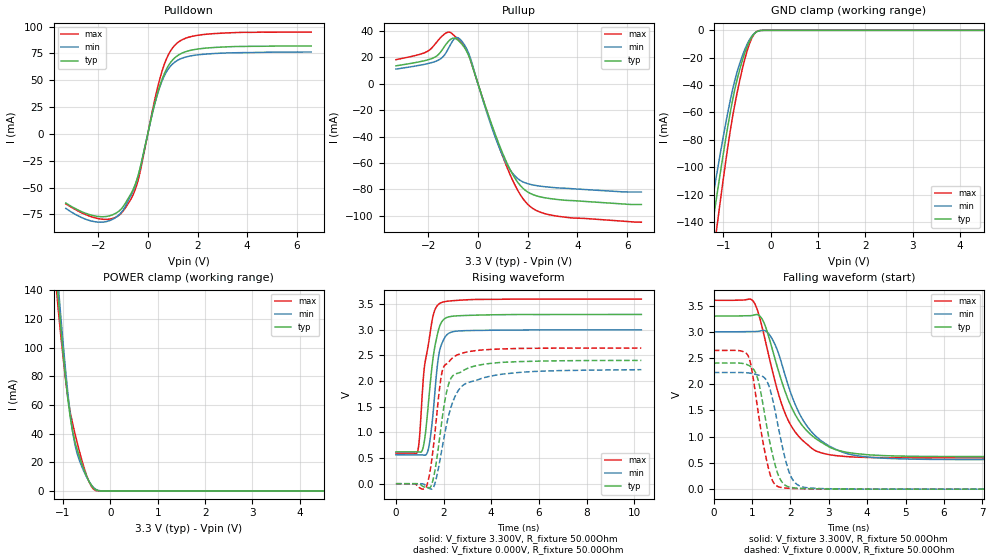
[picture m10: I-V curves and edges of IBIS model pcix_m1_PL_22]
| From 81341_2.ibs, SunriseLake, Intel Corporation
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[Model]   pcix_m1_PL_22
Model_type   I/O
Vinl = 1.155V
Vinh = 1.650V
Vmeas = 1.320V
Vref = 0.000V
Cref = 10.000pF
Rref = 25.000Ohm
|   typ   min   max
C_comp   7.500pF   6.000pF   9.000pF
[Voltage Range]   3.300V   3.000V   3.600V
[Temperature Range]   60.0   110.0   -5.0
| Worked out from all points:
|   slope of the pulldown table from 0 to 0.495 V, typ, clamps not added: 10.9 ohm
|   slope of the pullup table from 0 to 0.495 V, typ, clamps not added: 17.8 ohm
|   GND clamp passes 1 mA (typ) near -0.30 V on its own axis
|   POWER clamp passes 1 mA (typ) near -0.32 V on its own axis
|   falling waveform, V_fixture 3.300V, R_fixture 50.00Ohm: 20-80 % time 884ps typ, 883ps min, 737ps max; typ from 3.3 V to 0.62 V
|   rising waveform, V_fixture 3.300V, R_fixture 50.00Ohm: 20-80 % time 393ps typ, 315ps min, 421ps max; typ from 0.62 V to 3.3 V
|   rising waveform, V_fixture 0.000V, R_fixture 50.00Ohm: 20-80 % time 485ps typ, 727ps min, 388ps max; typ from 0 V to 2.4 V
|   falling waveform, V_fixture 0.000V, R_fixture 50.00Ohm: 20-80 % time 388ps typ, 399ps min, 356ps max; typ from 2.4 V to 0 V
[Pulldown]
|   Voltage   I(typ)   I(min)   I(max)
-3.3V     -64.47mA   -69.44mA   -65.21mA
-1.9V     -77.17mA   -82.31mA   -79.35mA
-1.35V    -74.74mA   -78.78mA   -78.28mA
-950mV    -66.39mA   -69.46mA   -70.57mA
-600mV    -52.29mA   -53.64mA   -57.12mA
-400mV    -39.68mA   -40.38mA   -43.96mA
200mV     20.68mA    20.76mA    23.27mA
500mV     45.92mA    44.9mA     52.67mA
850mV     64.34mA    61.31mA    74.75mA
1.25V     73.73mA    69.22mA    85.88mA
2.65V     80.49mA    74.87mA    93.43mA
6.575V    81.96mA    76.32mA    94.87mA
[GND Clamp]
|   Voltage   I(typ)   I(min)   I(max)
-3.3V     -632.5mA   -564.4mA   -725.5mA
-1.325V   -165.6mA   -144.4mA   -196mA
-1.3V     -159.5mA   -139mA     -189mA
-1.25V    -147.6mA   -128.4mA   -175.3mA
-1.2V     -135.8mA   -118mA     -161.6mA
-1.125V   -118.5mA   -102.6mA   -141.4mA
-850mV    -59.64mA   -50.8mA    -72.97mA
-650mV    -28.41mA   -23.93mA   -36.31mA
-450mV    -8.219mA   -7.112mA   -10.14mA
-350mV    -2.584mA   -2.413mA   -2.802mA
-250mV    -331.3uA   -398.2uA   -220.5uA
6.575V    0A         0A         0A
[Pullup]
|   Voltage   I(typ)   I(min)   I(max)
-3.3V     13.5mA     11.03mA    18.15mA
-2.15V    17.38mA    14.64mA    23.38mA
-1.65V    21.08mA    17.31mA    31.67mA
-1.1V     33.54mA    29.73mA    38.7mA
-850mV    33.56mA    34.9mA     34.67mA
-500mV    26.01mA    27.99mA    26.71mA
500mV     -28.04mA   -29.95mA   -28.73mA
1V        -52.86mA   -54.63mA   -55.12mA
1.5V      -71.83mA   -70.04mA   -77.08mA
2V        -81.86mA   -75.62mA   -91.14mA
3.2V      -87.59mA   -78.79mA   -100.2mA
6.575V    -91.38mA   -81.92mA   -104.7mA
[POWER Clamp]
|   Voltage   I(typ)   I(min)   I(max)
-3.3V     1.109A     1.089A     1.13A
-1.125V   144.6mA    153.4mA    135.7mA
-1.1V     134.6mA    143.1mA    126.5mA
-1.075V   125mA      133.1mA    118mA
-900mV    64.86mA    68.99mA    65.55mA
-800mV    41.99mA    41.86mA    47.4mA
-750mV    34.63mA    32.54mA    40.32mA
-650mV    23.51mA    20.95mA    27.23mA
-500mV    10.16mA    9.585mA    10.63mA
-400mV    3.792mA    4.116mA    3.102mA
-300mV    590.1uA    959uA      205.5uA
6.575V    0A         0A         0A
[Ramp]
R_load = 50.00Ohm
|   typ   min   max
dV/dt_r   1.442V/484.758ps   1.334V/725.060ps   1.587V/387.232ps
dV/dt_f   1.608V/883.635ps   1.462V/882.649ps   1.803V/736.686ps
[Falling Waveform]
V_fixture = 3.300V
V_fixture_min = 3.000V
V_fixture_max = 3.600V
R_fixture = 50.00Ohm
|   Time   V(typ)   V(min)   V(max)
0s        3.3V       3V         3.6V
1.04ns    3.317V     3.004V     3.572V
1.25ns    3.254V     3.023V     3.119V
1.45ns    2.863V     2.947V     2.495V
1.88ns    1.822V     2.122V     1.41V
2.26ns    1.261V     1.403V     970.4mV
2.7ns     943mV      983mV      717.7mV
3.4ns     712.6mV    692.8mV    624.5mV
4.14ns    649.9mV    603.9mV    602.4mV
10.3ns    620.3mV    563mV      595.4mV
[Rising Waveform]
V_fixture = 3.300V
V_fixture_min = 3.000V
V_fixture_max = 3.600V
R_fixture = 50.00Ohm
|   Time   V(typ)   V(min)   V(max)
0s        620.3mV    563mV      595.4mV
900ps     620.3mV    562.4mV    612.8mV
990ps     617.2mV    562.7mV    905.6mV
1.12ns    667mV      561.2mV    1.855V
1.21ns    881.7mV    555.4mV    2.327V
1.41ns    1.804V     792.2mV    2.859V
1.6ns     2.58V      1.585V     3.342V
1.84ns    3.077V     2.606V     3.516V
2.57ns    3.273V     2.976V     3.575V
10.3ns    3.3V       3V         3.6V
[Rising Waveform]
V_fixture = 0.000V
V_fixture_min = 0.000V
V_fixture_max = 0.000V
R_fixture = 50.00Ohm
|   Time   V(typ)   V(min)   V(max)
0s        601.5nV    3.438uV    42.63nV
1.27ns    -72.21mV   -43.87mV   -65.04mV
1.56ns    80.99mV    -85.65mV   671mV
1.82ns    841.2mV    390.1mV    1.814V
1.94ns    1.267V     698.5mV    2.187V
2.2ns     1.924V     1.304V     2.361V
2.5ns     2.139V     1.72V      2.494V
2.95ns    2.238V     1.957V     2.565V
4.35ns    2.362V     2.128V     2.626V
10.3ns    2.404V     2.223V     2.645V
[Falling Waveform]
V_fixture = 0.000V
V_fixture_min = 0.000V
V_fixture_max = 0.000V
R_fixture = 50.00Ohm
|   Time   V(typ)   V(min)   V(max)
0s        2.404V     2.223V     2.645V
900ps     2.363V     2.215V     2.535V
990ps     2.318V     2.206V     2.286V
1.14ns    2.12V      2.178V     1.555V
1.38ns    1.205V     2.064V     544.4mV
1.52ns    697.4mV    1.758V     179.3mV
1.7ns     237.5mV    1.119V     42.69mV
2ns       35.15mV    260.3mV    14.72mV
2.37ns    12.48mV    33.69mV    6.082mV
10.3ns    601.5nV    3.438uV    42.63nV
